FUNCTION_BLOCK Example07_sun //4x3 flyways 2 xbots - sun planet
VAR_INPUT
	Execute : BOOL;
END_VAR
VAR_OUTPUT
	Done : BOOL;
END_VAR
VAR_IN_OUT
	PM_Controller : PMControllerType;	// the planar motor controller to use
END_VAR
VAR
	xbotID_array78 : ARRAY[0..77] OF USINT;
	PosX_array78 : ARRAY[0..77] OF REAL;
	PosY_array78 : ARRAY[0..77] OF REAL;
	PMC_AutoDrivingMotion1 : PMC_AutoDrivingMotion;
	xbotID_array32 : ARRAY[0..31] OF USINT;
	PMC_PlanetMotionCtrl1 : PMC_PlanetMotionCtrl;
	PMC_XYMotion1 : PMC_XYMotion;
	PMC_XYMotion2 : PMC_XYMotion;
	PMC_PlanetMotionCtrl2 : PMC_PlanetMotionCtrl;
	PMC_XYMotion3 : PMC_XYMotion;
	PMC_XYMotion4 : PMC_XYMotion;
END_VAR

//4x3 flyways 2 xbots - sun planet

//async move to 60,60 and 60,180
xbotID_array78[0] := 1;xbotID_array78[1] := 2;
PosX_array78[0] := 0.06;PosX_array78[1] := 0.06;
PosY_array78[0] := 0.06;PosY_array78[1] := 0.18;
PMC_AutoDrivingMotion1(Execute := Execute,nXbots := 2,XbotID := xbotID_array78,RoutingType := 0,ZoneID := 0,PosX := PosX_array78,PosY := PosY_array78,PM_Controller := PM_Controller);

//set xbot 2 as a planet to xbot 1
xbotID_array32[0] := 2;
PMC_PlanetMotionCtrl1(Execute := PMC_AutoDrivingMotion1.Done,Level := 1,StarXID := 1,nXbots := 1,PlanetXID := xbotID_array32,PM_Controller := PM_Controller);

//move xbot 1 to 900,60
PMC_XYMotion1(Execute := PMC_PlanetMotionCtrl1.Done,cmdLB := 3,XbotID := 1,Mode := 0,Type_ := 0,PosX := 0.9,PosY := 0.06,EndVel := 0,MaxVel := 1,MaxAcc := 10,PM_Controller := PM_Controller);

//move xbot 1 to 60,60
PMC_XYMotion2(Execute := PMC_XYMotion1.Done,cmdLB := 4,XbotID := 1,Mode := 0,Type_ := 0,PosX := 0.06,PosY := 0.06,EndVel := 0,MaxVel := 1,MaxAcc := 10,PM_Controller := PM_Controller);

//disconnect xbot 2 from xbot 1
xbotID_array32[0] := 2;
PMC_PlanetMotionCtrl2(Execute := PMC_XYMotion2.Done,Level := 0,StarXID := 1,nXbots := 1,PlanetXID := xbotID_array32,PM_Controller := PM_Controller);

//move xbot 1 to 900,60
PMC_XYMotion3(Execute := PMC_PlanetMotionCtrl2.Done,cmdLB := 6,XbotID := 1,Mode := 0,Type_ := 0,PosX := 0.9,PosY := 0.06,EndVel := 0,MaxVel := 1,MaxAcc := 10,PM_Controller := PM_Controller);

//move xbot 1 to 60,60
PMC_XYMotion4(Execute := PMC_XYMotion3.Done,cmdLB := 7,XbotID := 1,Mode := 0,Type_ := 0,PosX := 0.06,PosY := 0.06,EndVel := 0,MaxVel := 1,MaxAcc := 10,PM_Controller := PM_Controller);

Done := PMC_XYMotion4.Done;

END_FUNCTION_BLOCK
